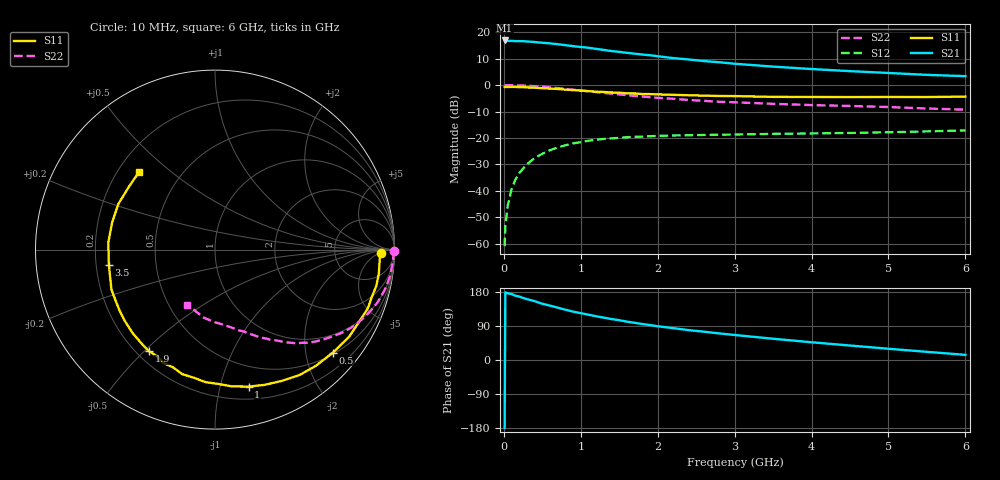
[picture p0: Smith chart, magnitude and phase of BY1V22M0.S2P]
! SIEMENS Small Signal Semiconductors
! BFY420
! Si NPN RF SIEGET Grounded Emitter Transistor in MICRO-X
! VCE = 1.25 V  IC = 2 mA
! Common Emitter S-Parameters:  October  1996
# GHz  S  MA  R  50
!  f  S11  S21  S12  S22
! GHz  MAG  ANG  MAG  ANG  MAG  ANG  MAG  ANG
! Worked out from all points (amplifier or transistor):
!   36 points, 10 MHz to 6 GHz, reference 50 ohm
!   highest |S21| = 16.9 dB at 10 MHz (marker M1)
!   |S21| within 3 dB of that: start of sweep to 1.154 GHz
!   unconditionally stable (mu >= 1): 3.985 GHz to end of sweep
!   at 250 MHz: K = 0.06, MSG = 24.1 dB, |S12| = -31.6 dB
!   at 1.4 GHz: K = 0.31, MSG = 16.5 dB, |S12| = -20.2 dB
!   at 6 GHz: K = 1.27, MAG = 7.2 dB, |S12| = -17.2 dB
!   S11 on the Smith chart (normalised r, x): 10 MHz: 23, -6; 500 MHz: 0.54, -2.57; 1 GHz: 0.31, -1.23; 1.9 GHz: 0.25, -0.52; 3.5 GHz: 0.25, -0.07; 6 GHz: 0.29, +0.39
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0.01  0.9224 -1.2  6.969 -179.6  0.0009 94.9  0.9968 -0.5
0.02  0.9197 -1.8  6.925 178.4  0.0022 92.4  0.9936 -0.9
0.05  0.9195 -4.4  6.808 176.3  0.0052 84.5  0.9948 -2.3
0.1  0.9227 -8.5  6.846 174.0  0.0106 85.9  0.9912 -4.6
0.15  0.9213 -12.6  6.768 169.7  0.0163 81.3  0.9882 -7.0
0.2  0.9125 -16.9  6.766 167.4  0.0215 81.4  0.9851 -9.1
0.25  0.9125 -20.9  6.766 163.9  0.0264 77.1  0.9779 -11.5
0.4  0.8911 -33.1  6.504 155.3  0.0416 70.7  0.9522 -18.0
0.5  0.8722 -41.1  6.305 148.4  0.0503 65.9  0.9283 -22.1
0.7  0.8428 -56.0  5.926 138.1  0.0663 57.5  0.8757 -29.7
0.9  0.8023 -70.0  5.437 127.8  0.079 50.3  0.8174 -36.1
1  0.7858 -76.2  5.247 123.6  0.0831 47.0  0.7887 -39.2
1.1  0.7681 -82.9  5.062 119.4  0.0886 44.0  0.762 -42.1
1.4  0.7238 -99.3  4.389 108.1  0.0982 36.1  0.69 -49.2
1.6  0.6963 -109.7  4.064 101.2  0.1032 32.0  0.6435 -53.2
1.9  0.6752 -123.1  3.656 92.2  0.1078 27.0  0.5899 -58.5
2.2  0.6537 -134.5  3.238 84.0  0.1114 22.7  0.5503 -62.9
2.8  0.6216 -153.7  2.697 70.2  0.1151 17.2  0.4829 -70.7
3.5  0.5974 -172.0  2.232 56.1  0.1195 13.1  0.4416 -78.5
4.5  0.5927 165.3  1.832 38.2  0.1244 9.3  0.4026 -91.1
5.5  0.5939 144.0  1.559 21.5  0.1331 7.0  0.3606 -107.2
6  0.605 134.4  1.473 13.6  0.1387 5.9  0.3422 -116.6
